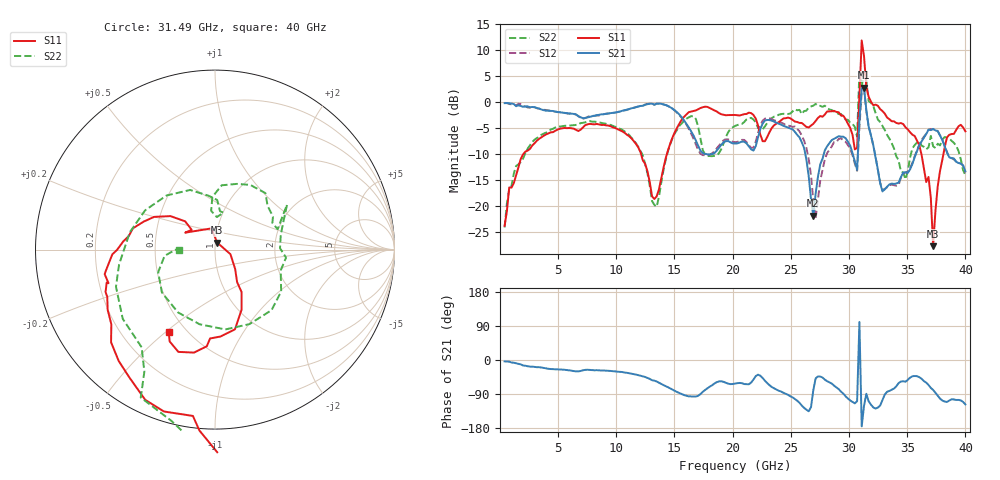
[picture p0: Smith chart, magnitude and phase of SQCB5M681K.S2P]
! Network Analyzer HP8722ES.07.66: Jul 25, 2000 Serial No. US39175408
! 27 Oct 2004  14:43:23
! Frequency  S11  S21  S12  S22
# HZ  S  DB R  50
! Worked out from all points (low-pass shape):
!   201 points, 400 MHz to 40 GHz, reference 50 ohm
!   highest |S21| = 2.79 dB at 31.29 GHz (marker M1); lowest = -21.8 dB at 26.93 GHz (marker M2)
!   |S21| within 3 dB of the highest: start of sweep to 685.4 MHz; 31 GHz to 31.43 GHz (429.4 MHz wide, 1.38 % of centre)
!   lowest |S11| = -27.7 dB at 37.23 GHz (marker M3), VSWR 1.09, Z = 51 + j4.04 ohm
!   |S11| at or under -10 dB: start of sweep to 2.005 GHz; 12.13 GHz to 14.34 GHz (2.217 GHz wide, 16.8 % of centre); 36.22 GHz to 38.11 GHz (1.89 GHz wide, 5.09 % of centre)
!   |S22| runs from -24.1 to 5.9 dB; largest |S21 - S12| = 0.15
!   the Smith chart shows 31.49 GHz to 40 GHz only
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4e8  -23.76 -106.5  -0.20 -3.7  -0.15 -3.2  -24.08 -105.0
2.776e9  -8.34 -103.8  -0.94 -17.4  -0.99 -17.6  -7.66 -111.7
7.132e9  -4.88 -99.1  -3.09 -27.2  -3.19 -28.0  -3.98 -124.0
1.3666e10  -16.75 -11.8  -0.29 -59.9  -0.29 -60.7  -18.16 58.0
1.6834e10  -1.59 1.0  -7.37 -96.4  -8.11 -96.8  -3.22 -66.3
2.02e10  -2.47 -0.9  -7.96 -62.2  -7.70 -61.5  -4.59 -15.2
2.515e10  -3.43 -9.5  -5.24 -98.7  -4.77 -101.2  -1.78 -17.3
2.614e10  -4.40 -79.8  -8.82 -126.3  -7.41 -126.5  -1.72 -13.6
2.6932e10  -4.16 -178.1  -21.83 -79.2  -18.94 -135.1  -0.67 -21.3
2.8318e10  -1.79 93.9  -7.86 -59.2  -9.16 -57.0  -1.43 -38.3
2.9704e10  -3.28 33.7  -6.93 -95.8  -7.61 -94.4  -3.35 -48.3
3.0694e10  -8.79 27.8  -12.99 -108.7  -13.21 -106.0  -6.65 -65.3
3.0892e10  1.24 15.1  -3.40 100.4  -4.88 109.5  5.85 -11.2
3.109e10  11.85 -66.8  2.64 -175.1  2.10 -172.5  3.00 137.7
3.1288e10  8.82 -83.4  2.79 -120.9  2.50 -118.5  5.72 -138.6
3.1486e10  2.96 -72.6  -1.50 -89.2  -1.69 -88.3  4.21 -93.8
3.1684e10  1.06 -89.4  -4.73 -108.8  -4.64 -108.5  0.21 -100.5
3.3466e10  -3.28 -150.8  -15.83 -81.6  -15.99 -82.2  -7.00 150.6
3.604e10  -8.29 151.7  -8.27 -45.4  -8.18 -45.7  -7.50 48.2
3.7228e10  -27.68 73.2  -5.16 -79.0  -5.19 -79.7  -8.49 13.1
3.8416e10  -6.78 -76.0  -9.68 -110.8  -9.56 -112.0  -6.79 -65.2
4e10  -5.60 -119.5  -13.31 -117.3  -13.51 -116.3  -14.03 -179.4
